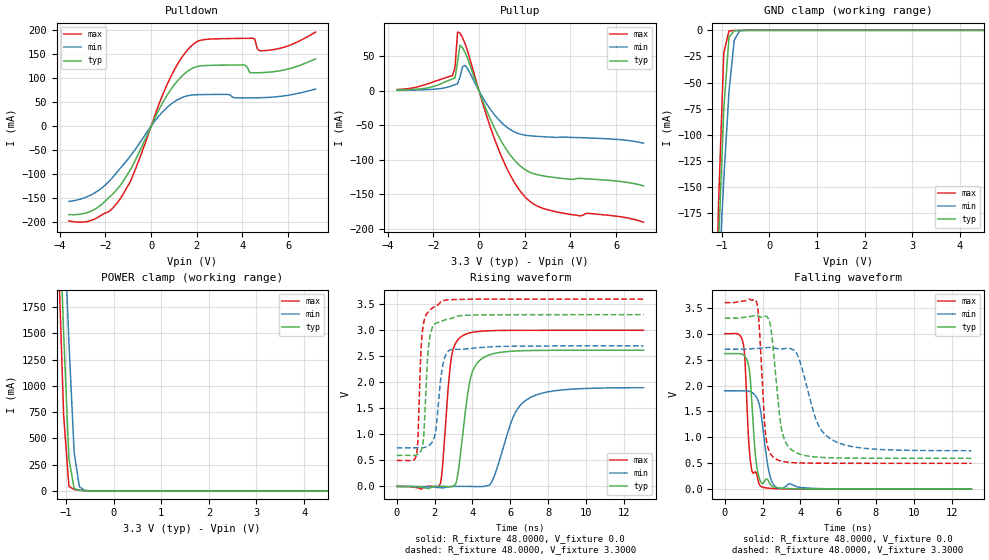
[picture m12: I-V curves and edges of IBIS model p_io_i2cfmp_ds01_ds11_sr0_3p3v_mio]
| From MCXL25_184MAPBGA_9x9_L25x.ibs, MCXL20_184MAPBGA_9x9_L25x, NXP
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[Model] p_io_i2cfmp_ds01_ds11_sr0_3p3v_mio
|   Model p_io_i2cfmp_ds01_ds11_sr0_3p3v_mio
| This model was characterised for following simulation conditions:
| External (pad) voltage:
|   - Typ: 3.3V,   - Min: 2.7V,   - Max: 3.6V
| Library cells for typ/min/max conditions are connected as defined below:
|  pad - External Pad
|  ipp_do_lv - Core Input
|  ipp_obe_lv - Output Buffer Enable
|  IOGC - NC
|  REFH3V3 - REFH3V3
|  REFL3V3 - REFL3V3
|  ZI - NC
|  abut_ncal_vddio[1] - vddio
|  abut_ncal_vddio[2] - vddio
|  abut_ncal_vddio[3] - vssio
|  abut_ncal_vddio[4] - vddio
|  abut_ncal_vddio[5] - vddio
|  abut_ncal_vddio[6] - vssio
|  abut_pcal_vddio[1] - vssio
|  abut_pcal_vddio[2] - vssio
|  abut_pcal_vddio[3] - vddio
|  abut_pcal_vddio[4] - vssio
|  abut_pcal_vddio[5] - vssio
|  abut_pcal_vddio[6] - vddio
|  ipp_do_1p8v - ipp_do_1p8v
|  ipp_dse_lv[0] - vdd_lv
|  ipp_dse_lv[1] - vdd_lv
|  ipp_eftd_lv - NC
|  ipp_ina_mux_vddio - NC
|  ipp_ina_mux_vddio[0] - NC
|  ipp_ina_mux_vddio[1] - NC
|  ipp_ina_r0_vddio - NC
|  ipp_ina_r0a_vddio - NC
|  ipp_ina_r0b_vddio - NC
|  ipp_ina_r0c_vddio - NC
|  ipp_ina_r0d_vddio - NC
|  ipp_ina_r0e_vddio - NC
|  ipp_ina_r0f_vddio - NC
|  ipp_ina_r300_vddio - NC
|  ipp_ina_r300a_vddio - NC
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Model_type I/O
Polarity   Non-Inverting
Enable   Active-High
Vinl =   0.9900V
Vinh =   2.3100V
Vmeas =  1.6500V
Cref =   30.0000pF
Rref =   1.0000M
Vref =   3.3000V
C_comp   1.7403pF   1.7015pF   1.7922pF
|C_comp_pullup   0.6932pF   0.7569pF   0.6560pF
|C_comp_pulldown   0.9338pF   0.9188pF   0.9329pF
[Model Spec]
| variable   typ   min   max
Vinh   2.3100V   1.8900V   2.5200V
Vinl   0.9900V   0.8100V   1.0800V
[Temperature Range]   25.0000   0.1250k   -40.0000
[Voltage Range]   3.3000V   2.7000V   3.6000V
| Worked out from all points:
|   slope of the pulldown table from 0 to 0.495 V, typ, clamps not added: 10.3 ohm
|   slope of the pullup table from 0 to 0.495 V, typ, clamps not added: 12 ohm
|   GND clamp passes 1 mA (typ) near -0.75 V on its own axis
|   POWER clamp passes 1 mA (typ) near -0.52 V on its own axis
|   rising waveform, R_fixture 48.0000, V_fixture 0.0: 20-80 % time 572ps typ, 1.12ns min, 390ps max; typ from 0 V to 2.62 V
|   rising waveform, R_fixture 48.0000, V_fixture 3.3000: 20-80 % time 253ps typ, 339ps min, 218ps max; typ from 0.595 V to 3.3 V
|   falling waveform, R_fixture 48.0000, V_fixture 0.0: 20-80 % time 303ps typ, 421ps min, 259ps max; typ from 2.62 V to 0 V
|   falling waveform, R_fixture 48.0000, V_fixture 3.3000: 20-80 % time 466ps typ, 1.02ns min, 289ps max; typ from 3.3 V to 0.595 V
[Pulldown]
|Voltage   I(typ)   I(min)   I(max)
-3.6V     -184.6mA   -157.2mA   -197.8mA
-2.5V     -174.4mA   -140.2mA   -194.6mA
-1.4V     -126.7mA   -90.76mA   -155mA
-850mV    -86.25mA   -58.63mA   -109.3mA
800mV     72.05mA    43.26mA    97.24mA
1.9V      122.8mA    65.52mA    173.1mA
4.1V      127.8mA    58.94mA    183.5mA
4.43V     111.5mA    59.09mA    183.8mA
4.54V     111.5mA    59.18mA    181.9mA
4.65V     111.6mA    59.29mA    161.7mA
5.09V     112.6mA    60.08mA    158.3mA
7.2V      140.6mA    77.33mA    196.5mA
[Pullup]
|Voltage   I(typ)   I(min)   I(max)
-3.6V     1.234mA    737.3uA    1.918mA
-1.16V    17.44mA    7.571mA    22.18mA
-1.05V    18.81mA    8.961mA    34.26mA
-940mV    42.21mA    10.4mA     85.31mA
-830mV    66.21mA    20.76mA    83.9mA
-720mV    62.74mA    35.25mA    76.97mA
-610mV    55.53mA    37mA       68.37mA
820mV     -63.53mA   -40.29mA   -82.06mA
1.48V     -97.81mA   -58.39mA   -129mA
2.03V     -114.5mA   -64.35mA   -154.4mA
3.46V     -126.4mA   -67.4mA    -176.1mA
7.2V      -137.9mA   -75.9mA    -190.6mA
[GND_clamp]
|Voltage   I(typ)   I(min)   I(max)
-3.6V     -4.377A    -3.283A    -5.855A
-1.18V    -351.7mA   -346.5mA   -367.9mA
-1.07V    -204.2mA   -241.2mA   -166.2mA
-960mV    -75.42mA   -142.6mA   -21.4mA
-850mV    -6.575mA   -58.21mA   -529.8uA
-740mV    -281.6uA   -9.383mA   -183.8uA
-630mV    -73.66uA   -605.1uA   -74.76uA
-410mV    -3.148uA   -9.219uA   -1.868uA
7.2V      0A         0A         0A
[POWER_clamp]
|Voltage   I(typ)   I(min)   I(max)
-3.6V     34.56A     31.8A      37.41A
-1.16V    2.902A     3.904A     2.233A
-1.05V    1.495A     2.658A     715.5mA
-940mV    310.6mA    1.419A     44.07mA
-830mV    22.38mA    368.3mA    13.28mA
-720mV    6.713mA    39.84mA    7.005mA
-610mV    2.702mA    5.591mA    2.612mA
7.2V      0A         0A         0A
[Ramp]
| variable   typ   min   max
dV/dt_r  1.5700/0.5718n   1.1386/1.1169n   1.8003/0.3899n
dV/dt_f  1.6228/0.4658n   1.1750/1.0174n   1.8605/0.2894n
R_load = 48.0000
[Rising Waveform]
R_fixture= 48.0000
V_fixture= 0.0
V_fixture_min= 0.0
V_fixture_max= 0.0
|time   V(typ)   V(min)   V(max)
0s        1.18nV     98.79nV    3.846nV
2.301ns   3.247mV    -25.56mV   50.03mV
2.878ns   -7.192mV   -963.7uV   2.456V
3.164ns   108.1mV    1.744mV    2.783V
3.467ns   936mV      1.808mV    2.893V
3.95ns    2.148V     -594.2uV   2.958V
4.676ns   2.494V     5.307mV    2.988V
6.207ns   2.601V     1.372V     2.999V
6.934ns   2.61V      1.68V      3V
13.05ns   2.617V     1.898V     3.001V
[Rising Waveform]
R_fixture= 48.0000
V_fixture= 3.3000
V_fixture_min= 2.7000
V_fixture_max= 3.6000
|time   V(typ)   V(min)   V(max)
0s        595.3mV    740.4mV    499.2mV
1.047ns   605.1mV    740.4mV    620.3mV
1.113ns   616.5mV    740.3mV    876mV
1.309ns   706.8mV    740.9mV    2.794V
1.422ns   957.3mV    745.4mV    3.141V
1.728ns   2.822V     794.9mV    3.378V
2.052ns   3.133V     1.049V     3.465V
2.369ns   3.175V     2.19V      3.557V
2.949ns   3.235V     2.634V     3.59V
13.05ns   3.3V       2.7V       3.6V
[Falling Waveform]
R_fixture= 48.0000
V_fixture= 0.0
V_fixture_min= 0.0
V_fixture_max= 0.0
|time   V(typ)   V(min)   V(max)
0s        2.617V     1.899V     3.001V
961.1ps   2.598V     1.9V       2.842V
1.07ns    2.562V     1.901V     2.496V
1.223ns   2.446V     1.897V     1.232V
1.434ns   1.685V     1.868V     368.1mV
1.655ns   552mV      1.789V     321.9mV
1.931ns   125.1mV    1.435V     51.37mV
2.358ns   123.3mV    307.2mV    17.72mV
2.8ns     27.89mV    26.03mV    8.711mV
13.05ns   1.639uV    28.05uV    214.2nV
[Falling Waveform]
R_fixture= 48.0000
V_fixture= 3.3000
V_fixture_min= 2.7000
V_fixture_max= 3.6000
|time   V(typ)   V(min)   V(max)
0s        3.3V       2.7V       3.6V
1.698ns   3.356V     2.716V     3.597V
2.163ns   3.338V     2.729V     1.054V
2.407ns   3.182V     2.738V     690.9mV
2.66ns    2.341V     2.72V      592.1mV
3.059ns   1.073V     2.705V     536.1mV
3.775ns   704.8mV    2.638V     508.9mV
4.898ns   618mV      1.282V     501.1mV
5.729ns   603.9mV    942.5mV    499.9mV
13.05ns   595.3mV    741.6mV    499.2mV
